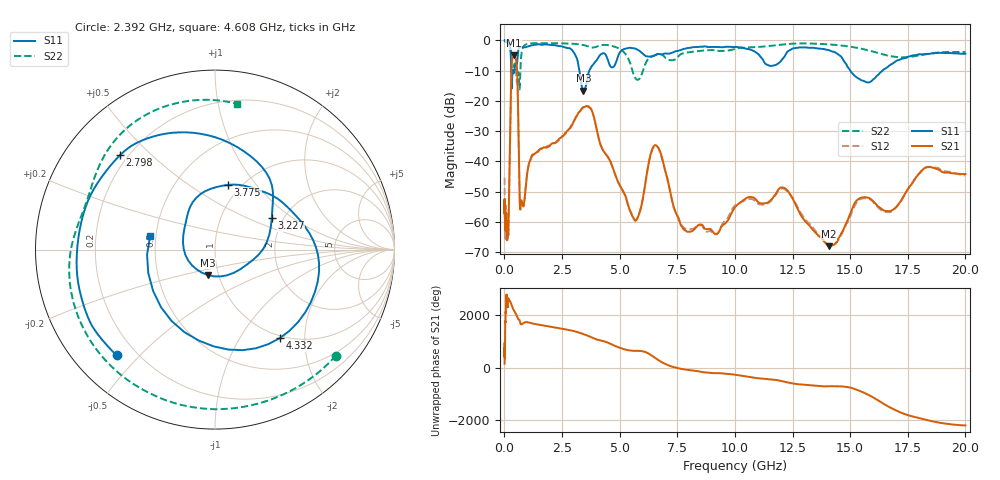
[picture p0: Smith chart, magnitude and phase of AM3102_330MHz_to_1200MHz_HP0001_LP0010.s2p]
! Date/Time: Tue, Sep 11, 2018 5:09 PM
! Network Analyzer: Agilent Technologies E8362B Rev: A.07.50.63
! Sweep from 0.010 to 20.000 GHz, 1601 Points, Sweep Type: LOG
! Power Supply: 4.950 V, 0.001 A
# Hz S DB R 50
!freq MagS11 AngS11 MagS21 AngS21 MagS12 AngS12 MagS22 AngS22
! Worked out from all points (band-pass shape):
!   1601 points, 10 MHz to 20 GHz, reference 50 ohm
!   highest |S21| = -4.87 dB at 406.7 MHz (marker M1); lowest = -68.0 dB at 14.07 GHz (marker M2)
!   |S21| within 3 dB of the highest: 317.7 MHz to 535.7 MHz (218 MHz wide, 51.1 % of centre)
!   lowest |S11| = -16.6 dB at 3.432 GHz (marker M3), VSWR 1.35, Z = 44.4 - j12.9 ohm
!   |S11| at or under -10 dB: 295.6 MHz to 357 MHz (61.35 MHz wide, 18.8 % of centre); 3.256 GHz to 3.681 GHz (425.9 MHz wide, 12.3 % of centre); 15.01 GHz to 16.4 GHz (1.393 GHz wide, 8.87 % of centre)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
!   |S22| runs from -16.2 to -0.2 dB; largest |S21 - S12| = 0.0082
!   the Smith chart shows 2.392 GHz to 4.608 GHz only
!   S11 on the Smith chart (normalised r, x): 2.392 GHz: 0.13, -0.43; 2.798 GHz: 0.17, +0.40; 3.227 GHz: 1.75, +0.70; 3.775 GHz: 0.87, +0.73; 4.332 GHz: 0.96, -1.51; 4.608 GHz: 0.46, +0.08
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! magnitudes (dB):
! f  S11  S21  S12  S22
! 10 MHz  0.0  -56.9  -45.4  -0.2
! 35.55 MHz  0.0  -62.2  -60.7  -0.4
! 126.4 MHz  -0.4  -63.4  -66.1  -0.8
! 182.2 MHz  -1.0  -59.8  -61.0  -1.2
! 406.7 MHz  -10.9  -4.9  -4.9  -8.7
! 447.2 MHz  -9.1  -5.3  -5.3  -7.6
! 559.1 MHz  -6.8  -11.2  -11.3  -13.5
! 685.8 MHz  -2.2  -55.7  -56.5  -12.2
! 1.59 GHz  -1.4  -35.7  -35.8  -0.9
! 2.392 GHz  -1.9  -32.3  -32.8  -1.0
! 2.798 GHz  -2.5  -29.3  -29.3  -1.0
! 3.227 GHz  -8.8  -23.8  -24.0  -1.3
! 3.432 GHz  -16.6  -22.0  -22.1  -1.5
! 3.775 GHz  -8.7  -22.8  -22.8  -2.3
! 4.332 GHz  -4.3  -36.9  -36.8  -1.5
! 4.608 GHz  -8.7  -40.1  -40.2  -1.7
! 5.652 GHz  -2.6  -59.4  -59.3  -12.1
! 6.58 GHz  -4.7  -34.7  -34.9  -4.8
! 7.882 GHz  -2.6  -63.0  -62.3  -4.0
! 12.09 GHz  -5.9  -48.6  -48.9  -1.3
! 14.07 GHz  -3.2  -68.0  -67.6  -1.3
! 20 GHz  -4.4  -44.2  -44.7  -3.8
